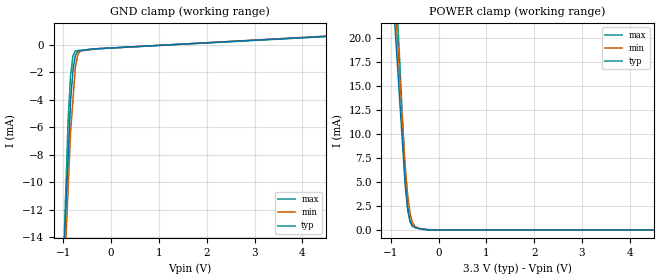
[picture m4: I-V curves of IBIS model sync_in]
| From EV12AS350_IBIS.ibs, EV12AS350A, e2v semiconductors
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[Model] sync_in
Model_type Input
Vinl = 1.15000V
Vinh = 1.35000V
C_comp 1.14000pF 1.09000pF 1.19000pF
| variable typ   min   max
[Voltage Range] 3.30000V 3.20000V 3.40000V
[POWER Clamp Reference] 3.30000V 3.20000V 3.40000V
[GND Clamp Reference] 0.00000V 0.00000V 0.00000V
[Temperature Range]   25   110   -40
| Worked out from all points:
|   GND clamp passes 1 mA (typ) near -0.76 V on its own axis
|   POWER clamp passes 1 mA (typ) near -0.60 V on its own axis
[GND Clamp]
-3.3V     -200.4mA   -203.3mA   -258.2mA
-900mV    -8.115mA   -10.41mA   -5.429mA
-850mV    -4.109mA   -6.39mA    -2.256mA
-800mV    -1.86mA    -4.017mA   -820.6uA
-750mV    -769.1uA   -1.644mA   -433uA
-700mV    -435.1uA   -735.4uA   -413.7uA
-650mV    -413.7uA   -445.6uA   -394.4uA
-375mV    -295.8uA   -306.9uA   -288.5uA
-350mV    -285uA     -294.3uA   -283.9uA
-325mV    -280.3uA   -281.7uA   -279.2uA
6.6V      1.027mA    1.053mA    1.004mA
[POWER Clamp]
-3.3V     205.9mA    215.9mA    275.1mA
-800mV    12.33mA    14.65mA    15.93mA
-700mV    4.588mA    6.596mA    5.56mA
-650mV    2.184mA    3.701mA    2.373mA
-600mV    906uA      1.77mA     876.8uA
-550mV    412.6uA    780.8uA    404.1uA
-500mV    246.2uA    404.3uA    313.1uA
-450mV    186.4uA    238.2uA    222uA
-175mV    0A         0A         13.1uA
6.6V      0A         0A         0A
